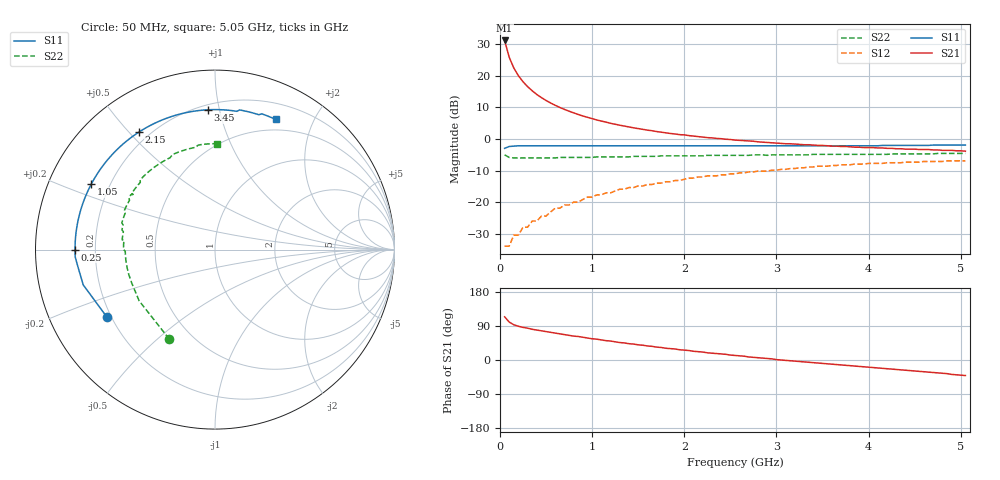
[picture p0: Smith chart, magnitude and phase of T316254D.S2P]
!AT-31625
!S-PARAMETERS at Vce=3.6 V  Ic=200 mA.  LAST UPDATED 08-05-96
# ghz s ma r 50
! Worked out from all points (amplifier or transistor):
!   101 points, 50 MHz to 5.05 GHz, reference 50 ohm
!   highest |S21| = 31.2 dB at 50 MHz (marker M1)
!   |S21| within 3 dB of that: start of sweep to 78.12 MHz
!   unconditionally stable (mu >= 1): 386.2 MHz to 441.4 MHz; 453.3 MHz to 1.969 GHz
!   at 850 MHz: K = 1.06, MAG = 12.3 dB, |S12| = -20.0 dB
!   at 2.55 GHz: K = 0.99, MSG = 5.4 dB, |S12| = -11.1 dB
!   at 5.05 GHz: K = 0.96, MSG = 1.5 dB, |S12| = -6.9 dB
!   S11 on the Smith chart (normalised r, x): 50 MHz: 0.18, -0.28; 250 MHz: 0.12, +0.00; 1.05 GHz: 0.13, +0.25; 2.15 GHz: 0.16, +0.53; 3.45 GHz: 0.23, +0.92; 5.05 GHz: 0.37, +1.50
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0.05  0.71 -148.0  36.39 114.0  0.02 41.0  0.56 -117.0
0.1  0.76 -165.0  19.69 100.0  0.02 43.0  0.51 -146.0
0.15  0.77 -173.0  13.31 93.0  0.03 49.0  0.5 -158.0
0.2  0.78 -177.0  10.04 89.0  0.03 54.0  0.5 -164.0
0.25  0.78 180.0  8.06 86.0  0.04 57.0  0.5 -168.0
0.3  0.78 177.0  6.74 84.0  0.04 60.0  0.5 -171.0
0.35  0.78 175.0  5.79 81.0  0.05 62.0  0.5 -173.0
0.4  0.78 173.0  5.06 79.0  0.05 63.0  0.5 -174.0
0.5  0.78 169.0  4.07 75.0  0.06 64.0  0.5 -177.0
0.55  0.78 167.0  3.71 73.0  0.07 64.0  0.5 -178.0
0.65  0.78 164.0  3.15 69.0  0.08 64.0  0.51 180.0
0.75  0.78 161.0  2.75 65.0  0.09 64.0  0.51 178.0
0.9  0.78 156.0  2.31 60.0  0.11 62.0  0.51 176.0
1.05  0.78 152.0  2 55.0  0.13 61.0  0.52 174.0
1.3  0.78 145.0  1.65 46.0  0.16 57.0  0.52 170.0
1.75  0.78 133.0  1.28 33.0  0.2 50.0  0.54 164.0
2.15  0.78 123.0  1.09 22.0  0.25 43.0  0.54 159.0
2.55  0.78 113.0  0.96 12.0  0.28 36.0  0.55 152.0
3.4  0.78 94.0  0.8 -7.0  0.36 20.0  0.57 137.0
3.45  0.78 93.0  0.79 -8.0  0.37 19.0  0.57 136.0
4.25  0.79 78.0  0.71 -24.0  0.42 2.0  0.58 114.0
5.05  0.8 65.0  0.64 -41.0  0.45 -15.0  0.59 89.0
